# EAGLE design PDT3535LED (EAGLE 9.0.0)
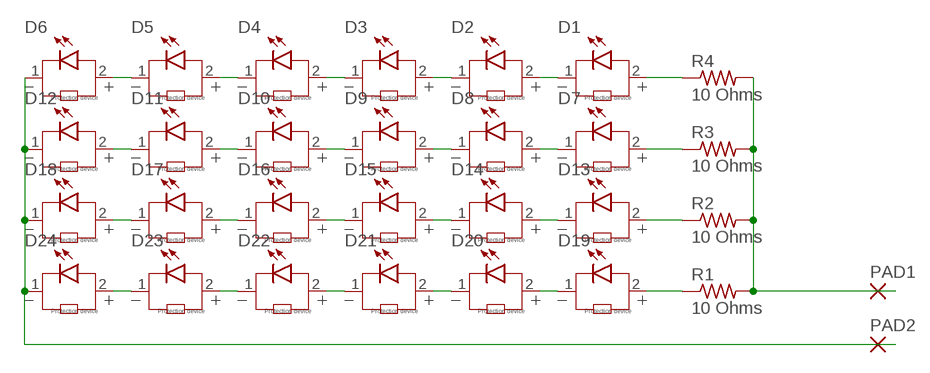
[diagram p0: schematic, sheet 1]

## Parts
D1  WL-SWTC_3535_158353060_6000K  [WL-SWTC_3535]
D2  WL-SWTC_3535_158353060_6000K  [WL-SWTC_3535]
D3  WL-SWTC_3535_158353060_6000K  [WL-SWTC_3535]
D4  WL-SWTC_3535_158353060_6000K  [WL-SWTC_3535]
D5  WL-SWTC_3535_158353060_6000K  [WL-SWTC_3535]
D6  WL-SWTC_3535_158353060_6000K  [WL-SWTC_3535]
D7  WL-SWTC_3535_158353060_6000K  [WL-SWTC_3535]
D8  WL-SWTC_3535_158353060_6000K  [WL-SWTC_3535]
D9  WL-SWTC_3535_158353060_6000K  [WL-SWTC_3535]
D10  WL-SWTC_3535_158353060_6000K  [WL-SWTC_3535]
D11  WL-SWTC_3535_158353060_6000K  [WL-SWTC_3535]
D12  WL-SWTC_3535_158353060_6000K  [WL-SWTC_3535]
D13  WL-SWTC_3535_158353060_6000K  [WL-SWTC_3535]
D14  WL-SWTC_3535_158353060_6000K  [WL-SWTC_3535]
D15  WL-SWTC_3535_158353060_6000K  [WL-SWTC_3535]
D16  WL-SWTC_3535_158353060_6000K  [WL-SWTC_3535]
D17  WL-SWTC_3535_158353060_6000K  [WL-SWTC_3535]
D18  WL-SWTC_3535_158353060_6000K  [WL-SWTC_3535]
D19  WL-SWTC_3535_158353060_6000K  [WL-SWTC_3535]
D20  WL-SWTC_3535_158353060_6000K  [WL-SWTC_3535]
D21  WL-SWTC_3535_158353060_6000K  [WL-SWTC_3535]
D22  WL-SWTC_3535_158353060_6000K  [WL-SWTC_3535]
D23  WL-SWTC_3535_158353060_6000K  [WL-SWTC_3535]
D24  WL-SWTC_3535_158353060_6000K  [WL-SWTC_3535]
PAD1  1,6/0,8  [1,6/0,8]
PAD2  1,6/0,8  [1,6/0,8]
R1  10 Ohms  R-US_0617/22  [0617/22]
R2  10 Ohms  R-US_0617/22  [0617/22]
R3  10 Ohms  R-US_0617/22  [0617/22]
R4  10 Ohms  R-US_0617/22  [0617/22]

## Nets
N$1: D19.2 R1.1
N$2: D19.1 D20.2
N$3: D20.1 D21.2
N$4: D21.1 D22.2
N$5: D22.1 D23.2
N$6: D23.1 D24.2
N$7: D13.2 R2.1
N$8: D13.1 D14.2
N$9: D14.1 D15.2
N$10: D15.1 D16.2
N$11: D16.1 D17.2
N$12: D17.1 D18.2
N$13: D7.2 R3.1
N$14: D7.1 D8.2
N$15: D8.1 D9.2
N$16: D9.1 D10.2
N$17: D10.1 D11.2
N$18: D11.1 D12.2
N$19: D1.2 R4.1
N$20: D1.1 D2.2
N$21: D2.1 D3.2
N$22: D3.1 D4.2
N$23: D4.1 D5.2
N$24: D5.1 D6.2
N$25: D6.1 D12.1 D18.1 D24.1 PAD2.1(P)
N$26: PAD1.1(P) R1.2 R2.2 R3.2 R4.2

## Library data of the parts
D1-D24 = Wurth_Elektronik_Optoelectronics_rev17b:WL-SWTC_3535: WL-SWTC
PAD1 PAD2 = wirepad:1,6/0,8: THROUGH-HOLE PAD
R1-R4 = resistor:R-US_: RESISTOR, American symbol

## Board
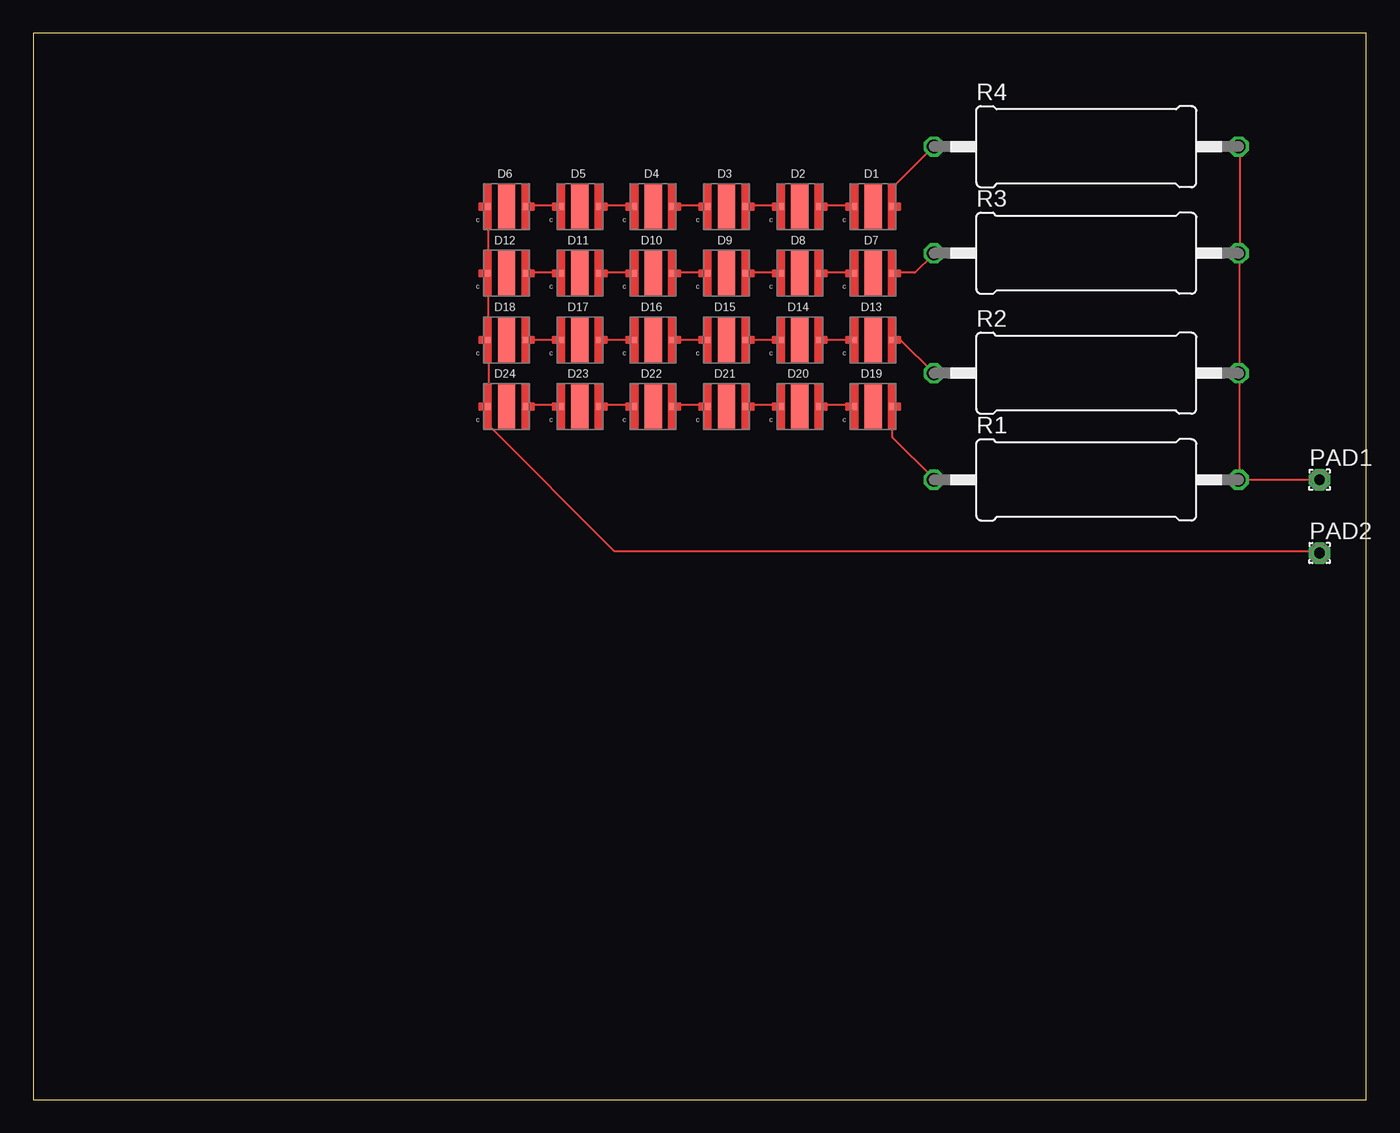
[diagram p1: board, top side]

Size 100 x 80 mm. Coordinates in mm from the lower left corner, seen from the top.
Outline: 0,0 100,0 100,80 0,80 0,0
Copper layers (1*16): Top 0.035mm / dielectric 1.5mm / Bottom 0.035mm
Design rules "default": minimum track width 6mil, minimum drill 0.35mm, track to track 6mil, track to pad 6mil, pad to pad 6mil, via to via 6mil, smd to smd 6mil, copper to edge 40mil, drill to drill 6mil, minimum pad ring 10mil, minimum via ring 8mil, stop-mask expansion 4mil, vias tented up to drill 0mil, thermal gap 10mil

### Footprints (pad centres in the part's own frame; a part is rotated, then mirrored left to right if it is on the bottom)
WL-SWTC_3535 = smd 0.4 x 0.5: 1 -1.4,0; 2 1.4,0 | smd 1.3 x 3.3: 3 0,0
1,6/0,8 = drill 0.813 pad 1.6 octagon: 1 0,0
0617/22 = drill 1.016 octagon: 1 -11.43,0; 2 11.43,0

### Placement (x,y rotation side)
D1  63,67 0 top
D2  57.5,67 0 top
D3  52,67 0 top
D4  46.5,67 0 top
D5  41,67 0 top
D6  35.5,67 0 top
D7  63,62 0 top
D8  57.5,62 0 top
D9  52,62 0 top
D10  46.5,62 0 top
D11  41,62 0 top
D12  35.5,62 0 top
D13  63,57 0 top
D14  57.5,57 0 top
D15  52,57 0 top
D16  46.5,57 0 top
D17  41,57 0 top
D18  35.5,57 0 top
D19  63,52 0 top
D20  57.5,52 0 top
D21  52,52 0 top
D22  46.5,52 0 top
D23  41,52 0 top
D24  35.5,52 0 top
PAD1  96.5,46.5 0 top
PAD2  96.5,41 0 top
R1  79,46.5 0 top
R2  79,54.5 0 top
R3  79,63.5 0 top
R4  79,71.5 0 top

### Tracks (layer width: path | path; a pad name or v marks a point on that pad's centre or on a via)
N$1
  Top 0.152: D19.2 64.47,51.97 64.47,49.68 67.51,46.63 R1.1
N$2
  Top 0.152: D20.2 58.98,52.12 61.57,52.12 D19.1
N$3
  Top 0.152: D21.2 53.49,52.12 56.08,52.12 D20.1
N$4
  Top 0.152: D22.2 48.01,52.12 50.6,52.12 D21.1
N$5
  Top 0.152: D23.2 42.52,52.12 44.96,52.12 D22.1
N$6
  Top 0.152: D24.2 37.03,52.12 39.47,52.12 D23.1
N$7
  Top 0.152: D13.2 64.47,57 65.08,57 67.51,54.56 R2.1
N$8
  Top 0.152: D14.2 58.98,57 61.57,57 D13.1
N$9
  Top 0.152: D15.2 53.49,57 56.08,57 D14.1
N$10
  Top 0.152: D16.2 48.01,57 D15.1
N$11
  Top 0.152: D17.2 42.52,57 44.96,57 D16.1
N$12
  Top 0.152: D18.2 37.03,57 39.47,57 D17.1
N$13
  Top 0.152: D7.2 64.47,62.03 66.14,62.03 67.51,63.4 R3.1
N$14
  Top 0.152: D8.2 58.98,62.03 61.57,62.03 D7.1
N$15
  Top 0.152: D9.2 53.49,62.03 56.08,62.03 D8.1
N$16
  Top 0.152: D10.2 48.01,62.03 50.6,62.03 D9.1
N$17
  Top 0.152: D11.2 42.52,62.03 44.96,62.03 D10.1
N$18
  Top 0.152: D12.2 37.03,62.03 39.47,62.03 D11.1
N$19
  Top 0.152: D1.2 64.47,67.06 64.47,68.43 67.51,71.48 R4.1
N$20
  Top 0.152: D2.2 58.98,67.06 61.57,67.06 D1.1
N$21
  Top 0.152: D3.2 53.49,67.06 56.08,67.06 D2.1
N$22
  Top 0.152: D4.2 48.01,67.06 50.6,67.06 D3.1
N$23
  Top 0.152: D5.2 42.52,67.06 44.96,67.06 D4.1
N$24
  Top 0.152: D6.2 37.03,67.06 39.47,67.06 D5.1
N$25
  Top 0.152: D6.1 34.14,66.9 34.14,62.03 D12.1 34.14,61.87 34.14,57.15 D18.1 34.14,57 34.14,52.12 D24.1 34.14,51.97 34.14,50.6 43.59,41.15 96.47,41.15 PAD2.1
N$26
  Top 0.152: R4.2 90.53,71.48 90.53,63.55 R3.2 90.53,63.4 90.53,54.56 R2.2 90.53,54.41 90.53,46.63 | 90.53,46.63 R1.2 | PAD1.1 90.66,46.5 90.53,46.63

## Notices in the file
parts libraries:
Wurth_Elektronik_Optoelectronics_rev17b: Copyright: Würth Elektronik
